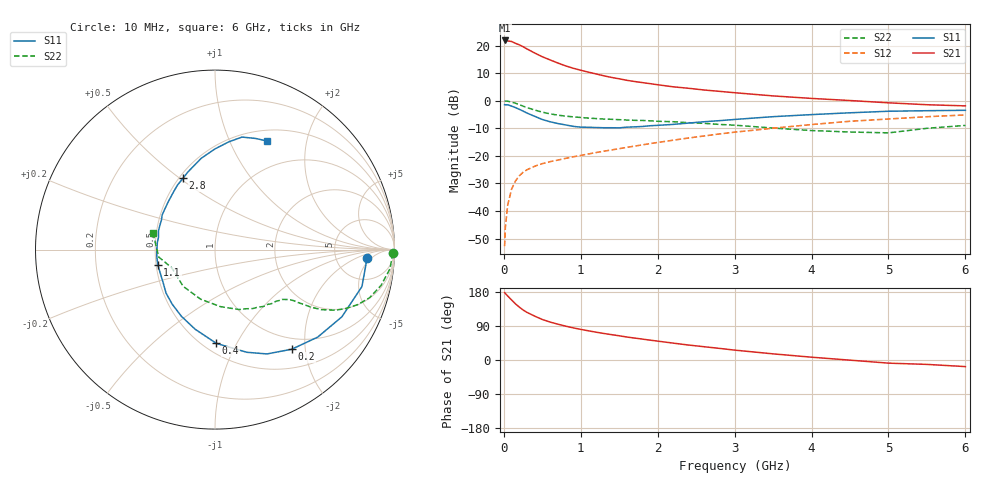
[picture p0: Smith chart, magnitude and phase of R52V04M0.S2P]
! SIEMENS Small Signal Semiconductors
! BFR183
! Si NPN RF Bipolar Junction Transistor in SOT23
! VCE = 2 V  IC = 4 mA
! Common Emitter S-Parameters:  May  1996
# GHz  S  MA  R  50
!  f  S11  S21  S12  S22
! GHz  MAG  ANG  MAG  ANG  MAG  ANG  MAG  ANG
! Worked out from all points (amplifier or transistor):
!   36 points, 10 MHz to 6 GHz, reference 50 ohm
!   highest |S21| = 21.9 dB at 10 MHz (marker M1)
!   |S21| within 3 dB of that: start of sweep to 295.9 MHz
!   unconditionally stable (mu >= 1): 1.132 GHz to 2.696 GHz
!   at 250 MHz: K = 0.36, MSG = 22.8 dB, |S12| = -26.0 dB
!   at 1.4 GHz: K = 1.06, MAG = 11.6 dB, |S12| = -17.9 dB
!   at 6 GHz: K = 0.90, MSG = 1.6 dB, |S12| = -5.1 dB
!   S11 on the Smith chart (normalised r, x): 10 MHz: 11, -3; 200 MHz: 0.80, -1.75; 400 MHz: 0.58, -0.83; 1.1 GHz: 0.51, -0.10; 2.8 GHz: 0.52, +0.51; 6 GHz: 0.63, +1.39
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0.01  0.8474 -3.0  12.41 178.0  0.0023 87.7  0.9934 -1.2
0.02  0.8449 -5.8  12.24 175.4  0.0051 86.7  0.9872 -2.6
0.05  0.8442 -14.1  12.18 169.0  0.0128 82.8  0.9806 -6.3
0.1  0.8 -27.9  11.89 158.6  0.0248 75.0  0.9462 -12.2
0.15  0.7519 -40.4  11.03 148.3  0.0348 69.2  0.902 -17.3
0.2  0.7006 -52.4  10.35 139.8  0.0434 65.0  0.8519 -21.1
0.25  0.6495 -63.5  9.564 132.0  0.0503 60.7  0.7982 -24.3
0.3  0.5989 -72.8  8.718 125.7  0.0558 58.3  0.7516 -26.7
0.4  0.5224 -89.2  7.363 115.9  0.0648 54.2  0.6792 -29.5
0.5  0.4569 -104.1  6.286 106.9  0.0722 52.5  0.621 -31.0
0.6  0.4161 -116.7  5.507 100.2  0.0785 51.9  0.5784 -31.8
0.7  0.3865 -128.1  4.849 94.6  0.0838 52.1  0.5489 -32.5
0.9  0.3432 -147.2  3.895 84.9  0.0961 52.6  0.5105 -33.4
1.1  0.3299 -165.4  3.301 77.0  0.1083 53.9  0.4848 -35.0
1.3  0.3237 179.8  2.835 70.0  0.1216 55.2  0.4658 -36.6
1.6  0.3318 161.6  2.348 60.6  0.1429 56.0  0.4463 -40.1
2.2  0.3722 134.5  1.79 44.6  0.1923 55.5  0.4165 -49.5
2.8  0.4353 114.2  1.482 30.7  0.2496 52.0  0.372 -62.4
3.5  0.5143 98.6  1.224 16.2  0.3175 45.2  0.3195 -84.4
4.5  0.6046 82.8  1.009 -0.4  0.4244 33.1  0.2708 -130.9
5.5  0.6596 69.8  0.847 -11.6  0.5129 20.2  0.3162 -172.5
6  0.671 64.4  0.807 -17.4  0.553 11.8  0.3569 165.2
